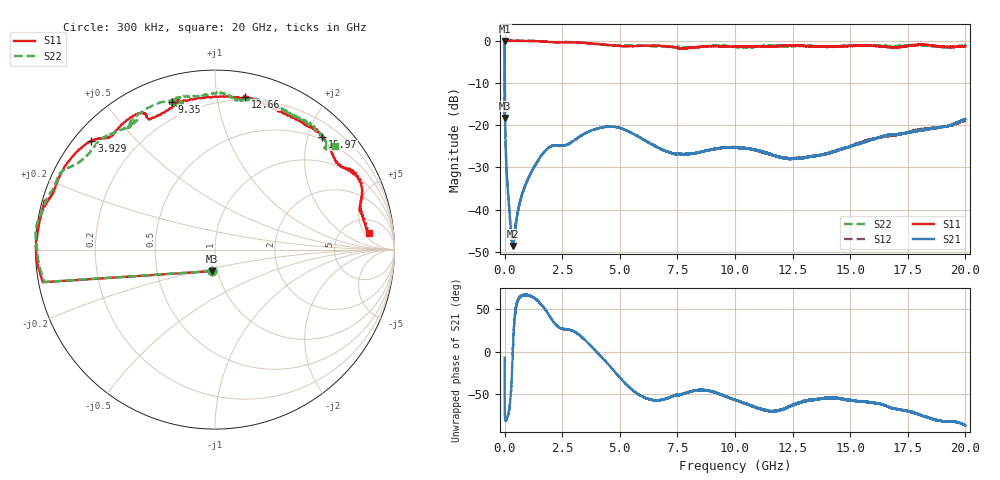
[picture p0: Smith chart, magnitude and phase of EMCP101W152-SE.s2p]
!EMCP101W152
!Johanson Technology Inc.
!www.johansontechnology.com
!Test Board Conditions:
!Substrate Type  RO4350B
!Substrate Thickness  10 mil
!Substrate Dk  3.66
!TL Type: GCPW
!TL Trace Width  20 mil
!TL Gap  10 mil
!PART MODE SINGLE ENDED (AKA BYPASS)
!DUT TOPOLOGY	SERIES-SHUNT
# MHz S  dB  R 50
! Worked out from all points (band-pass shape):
!   20001 points, 300 kHz to 20 GHz, reference 50 ohm
!   highest |S21| = -0.08 dB at 300 kHz (marker M1); lowest = -48.6 dB at 351.3 MHz (marker M2)
!   |S21| within 3 dB of the highest: start of sweep to 2.476 MHz
!   lowest |S11| = -18.3 dB at 300 kHz (marker M3), VSWR 1.28, Z = 46.9 - j11.4 ohm
!   |S11| at or under -10 dB: start of sweep to 1.016 MHz
!   |S22| runs from -18.4 to 0.0 dB; largest |S21 - S12| = 0.0058
!   S11 on the Smith chart (normalised r, x): 300 kHz: 0.94, -0.23; 3.929 GHz: 0.05, +0.38; 9.35 GHz: 0.12, +0.74; 12.66 GHz: 0.18, +1.20; 15.97 GHz: 0.46, +2.25; 20 GHz: 9, +6
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0.3  -18.30 -98.6  -0.08 -6.9  -0.08 -7.1  -18.37 -98.3
102.298  -0.01 -179.7  -32.14 -78.4  -32.11 -78.5  -0.08 -179.2
134.298  -0.03 179.7  -34.90 -76.0  -34.84 -75.9  -0.08 -179.8
258.296  -0.03 177.7  -43.82 -54.1  -43.91 -53.6  -0.05 178.6
351.295  -0.05 176.3  -48.63 -1.2  -48.55 -3.4  -0.02 177.9
816.288  -0.09 170.9  -35.44 66.3  -35.44 66.3  0.03 173.5
1572.276  -0.20 165.3  -27.38 55.8  -27.33 56.1  -0.17 163.7
3334.25  -0.48 145.8  -22.45 17.6  -22.47 17.6  -0.48 151.7
3929.241  -0.76 138.7  -20.98 1.9  -20.97 1.8  -0.82 148.6
5012.225  -1.27 133.9  -20.67 -30.4  -20.73 -30.5  -1.08 139.8
6667.2  -1.20 119.3  -25.38 -57.0  -25.29 -57.1  -1.38 129.6
7600.186  -1.81 115.3  -26.83 -50.6  -26.86 -50.4  -1.48 121.2
8631.171  -1.38 103.9  -26.19 -44.8  -26.19 -45.2  -1.42 123.9
9350.16  -1.33 106.2  -25.45 -49.5  -25.48 -49.0  -1.17 111.1
10000.15  -1.44 105.0  -25.33 -56.3  -25.19 -55.8  -1.48 102.9
11341.13  -1.31 79.4  -26.47 -68.5  -26.63 -68.8  -1.22 105.5
12655.11  -1.24 78.9  -27.89 -61.1  -27.80 -61.1  -1.21 92.3
13334.1  -1.36 71.7  -27.35 -56.3  -27.29 -57.0  -1.27 85.5
14359.08  -1.34 56.5  -26.13 -54.4  -26.17 -53.8  -1.43 79.2
15973.06  -1.27 46.4  -23.43 -59.5  -23.28 -60.9  -1.28 64.6
16667.05  -1.54 37.7  -22.27 -64.5  -22.56 -64.7  -1.25 62.8
20000  -1.32 6.2  -18.57 -86.2  -18.87 -84.7  -1.01 40.8
